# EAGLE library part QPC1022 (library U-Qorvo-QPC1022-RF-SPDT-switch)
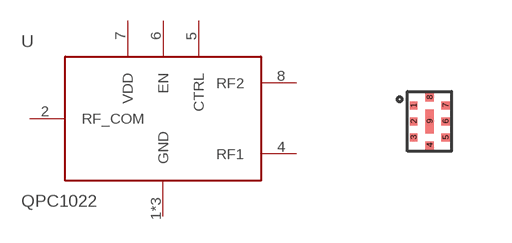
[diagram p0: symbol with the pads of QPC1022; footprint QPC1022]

Designator prefix U

## QPC1022 (MFR: Qorvo; MPN: QPC1022)  [QPC1022]
1  GND  pwr
2  RF_COM
3  GND  pwr
4  RF1
5  CTRL
6  EN
7  VDD  pwr
8  RF2
9  GND  pwr

## Footprint QPC1022 (pad centres in mm)
smd 0.2 x 0.2: 1 -0.4,0.4; 2 -0.4,0; 3 -0.4,-0.4; 4 0,-0.6; 5 0.4,-0.4; 6 0.4,0; 7 0.4,0.4; 8 0,0.6
smd 0.2 x 0.6: 9 0,0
